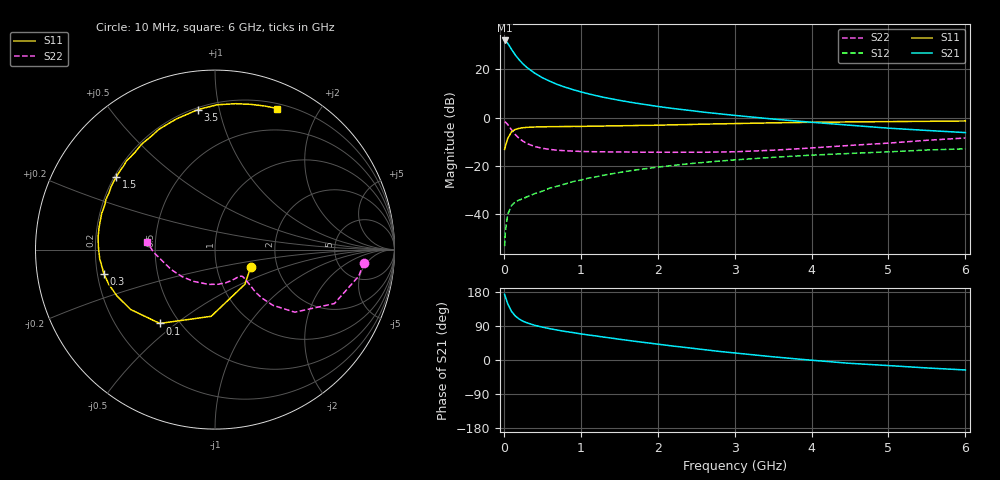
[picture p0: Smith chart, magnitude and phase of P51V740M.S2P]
! SIEMENS Small Signal Semiconductors
! BFP183
! Si NPN RF Bipolar Junction Transistor in SOT143
! VCE = 1.75 V  IC = 40 mA
! Common Emitter S-Parameters:  March  1996
# GHz  S  MA  R  50
!  f  S11  S21  S12  S22
! GHz  MAG  ANG  MAG  ANG  MAG  ANG  MAG  ANG
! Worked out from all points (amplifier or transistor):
!   36 points, 10 MHz to 6 GHz, reference 50 ohm
!   highest |S21| = 32.0 dB at 10 MHz (marker M1)
!   |S21| within 3 dB of that: start of sweep to 86.45 MHz
!   unconditionally stable (mu >= 1): start of sweep to 17.62 MHz; 290.8 MHz to end of sweep
!   at 250 MHz: K = 0.93, MSG = 27.9 dB, |S12| = -33.5 dB
!   at 1.4 GHz: K = 1.48, MAG = 11.4 dB, |S12| = -23.2 dB
!   at 6 GHz: K = 1.16, MAG = 1.0 dB, |S12| = -12.8 dB
!   S11 on the Smith chart (normalised r, x): 10 MHz: 1.46, -0.31; 100 MHz: 0.39, -0.44; 300 MHz: 0.23, -0.10; 1.5 GHz: 0.21, +0.32; 3.5 GHz: 0.21, +0.86; 6 GHz: 0.25, +1.51
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0.01  0.2224 -26.6  39.9 173.2  0.0022 75.8  0.8319 -5.0
0.02  0.255 -49.3  39.32 166.7  0.0044 74.1  0.8148 -10.4
0.05  0.3724 -93.3  35 148.5  0.01 67.0  0.73 -24.3
0.1  0.5136 -126.8  26.08 128.2  0.0153 51.9  0.5651 -38.1
0.15  0.5764 -144.6  19.9 115.8  0.0182 48.2  0.4475 -43.9
0.2  0.6044 -154.8  15.83 108.0  0.0199 47.5  0.3731 -46.0
0.25  0.6231 -162.1  13.01 102.3  0.0212 47.9  0.3269 -46.4
0.3  0.6335 -167.8  11.02 98.2  0.0231 50.0  0.293 -45.8
0.4  0.6444 -175.5  8.407 91.6  0.0269 52.3  0.2549 -44.9
0.5  0.65 178.6  6.764 86.8  0.0302 54.2  0.2336 -44.3
0.6  0.655 173.8  5.697 82.5  0.0352 56.5  0.2213 -44.2
0.7  0.6575 169.3  4.864 78.8  0.0386 58.2  0.2129 -44.5
0.8  0.6591 165.7  4.284 75.3  0.0428 58.7  0.2078 -45.3
1  0.6624 158.3  3.442 69.0  0.0514 59.6  0.2011 -48.2
1.1  0.6687 155.3  3.138 66.0  0.0564 59.2  0.1994 -49.9
1.5  0.6829 143.6  2.301 54.8  0.0737 58.0  0.1959 -58.4
2.2  0.7157 124.7  1.558 36.8  0.1033 52.1  0.193 -78.4
2.8  0.7479 110.5  1.211 22.7  0.1268 46.2  0.1961 -98.7
3.5  0.7858 97.0  0.941 8.4  0.1518 39.3  0.2132 -123.7
4.5  0.8211 81.9  0.701 -8.8  0.1829 29.3  0.268 -155.4
5.5  0.846 71.1  0.547 -21.0  0.2153 20.3  0.3423 -177.5
6  0.8594 66.1  0.494 -26.3  0.2279 15.2  0.382 173.4
